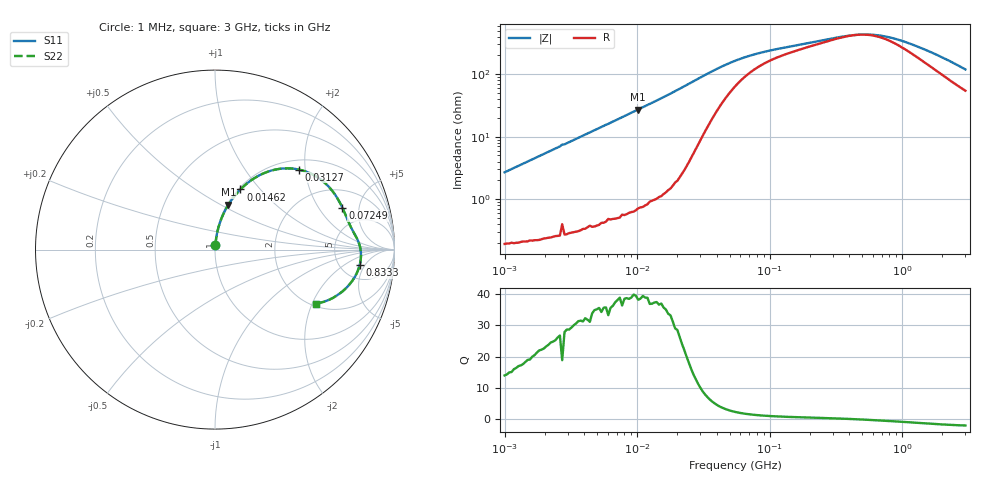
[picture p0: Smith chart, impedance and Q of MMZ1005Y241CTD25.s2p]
! S-Parameter Data Generated by TDK Corporation
! Copyright(C) 2025 TDK Corporation.
! All Rights Reserved.
! TDK P/N: MMZ1005Y241CTD25 (Chip Bead)
! Property: |Z|=240ohm at 100MHz
! Size(LxWxT): 1x0.5x0.5mm
! Model Type: s2p (Touchstone File Format Version 1.0)
! Frequency: DC=Yes Start=1MHz Stop=3000MHz 202points Log-sweep
! Model Generated on Feb. 6, 2025
! Terms and conditions regarding TDK Simulation Models:
! 1)This simulation model is being provided solely for informational
!  purposes. Please refer to the specifications of the products in
!  terms of detailed characteristics of such products.
! 2)In no event shall TDK Corporation of any of its subsidiaries be
!  liable for any loss or damage arising, directly or indirectly,
!  from any information contained in this simulation model, including,
!  but not limited to loss or damages arising from any inaccuracies,
!  omissions or errors in connection with such information.
! 3)Any and all copyrights on this simulation model are owned by
!  TDK Corporation.  Duplication or redistribution of this simulation
!  model without prior written permission from TDK Corporation
!  is prohibited.
! 4)This simulation model is subject to any modification or change
!  without any prior notice.
! 5)Neither TDK Corporation nor any of its subsidiaries shall make any
!  warranty, express or implied, including but not limited to the
!  correctness, implied warranties of merchantability and fitness for
!  a particular purpose with respect to this simulation models.
! 6)The use of this simulation model shall be deemed to have consented
!  to the terms and conditions hereof.
! Port Assignments:
!  1 ---@@@--- 2
! Applicable Conditions:
!  Temperature = 25 degC
!  DC Bias Current = 0 A
!  Small Signal Operation
# Hz S MA R 50
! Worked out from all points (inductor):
!   201 points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, 1 MHz to 3 GHz, reference 50 ohm
!   read as one part in series: L = 426 nH near 1.041 MHz
!   highest Q = 39.3 at 10.19 MHz (marker M1), where L = 425 nH
!   self-resonance near 467 MHz
!   S11 on the Smith chart (normalised r, x): 1 MHz: 1.00, +0.05; 14.62 MHz: 1.02, +0.79; 31.27 MHz: 1.21, +1.85; 72.49 MHz: 3.19, +3.37; 833.3 MHz: 7.61, -3.83; 3 GHz: 2.09, -2.12
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1000000  0.02679 84.4  0.9977 -1.5  0.9977 -1.5  0.02679 84.4
2055611  0.0547 84.4  0.9962 -3.1  0.9962 -3.1  0.0547 84.4
3900413  0.1031 82.3  0.9914 -5.9  0.9914 -5.9  0.1031 82.3
6058321  0.1575 79.2  0.9828 -9.1  0.9828 -9.1  0.1575 79.2
1.019448e7  0.2608 73.4  0.9586 -15.1  0.9586 -15.1  0.2608 73.4
1.461624e7  0.3638 67.1  0.9216 -21.3  0.9216 -21.3  0.3638 67.1
1.858443e7  0.4498 61.4  0.8788 -26.7  0.8788 -26.7  0.4498 61.4
2.362996e7  0.5453 54.1  0.8114 -33.0  0.8114 -33.0  0.5453 54.1
3.127247e7  0.6458 43.7  0.6948 -39.9  0.6948 -39.9  0.6458 43.7
4.138676e7  0.7086 33.1  0.5612 -43.6  0.5612 -43.6  0.7086 33.1
5.477226e7  0.7361 24.4  0.4488 -42.7  0.4488 -42.7  0.7361 24.4
7.248696e7  0.7472 18.2  0.3719 -38.8  0.3719 -38.8  0.7472 18.2
1.125904e8  0.759 11.9  0.3011 -31.3  0.3011 -31.3  0.759 11.9
2.136344e8  0.7824 6.4  0.239 -21.4  0.239 -21.4  0.7824 6.4
4.75755e8  0.8114 -0.2  0.1886 0.7  0.1886 0.7  0.8114 -0.2
6.049187e8  0.8141 -2.5  0.1901 10.9  0.1901 10.9  0.8141 -2.5
8.005644e8  0.8118 -5.6  0.208 22.5  0.208 22.5  0.8118 -5.6
8.332625e8  0.8107 -6.1  0.2122 24.0  0.2122 24.0  0.8107 -6.1
1.194682e9  0.7945 -10.9  0.266 34.3  0.266 34.3  0.7945 -10.9
1.645649e9  0.7643 -16.0  0.3385 38.4  0.3385 38.4  0.7643 -16.0
2.177892e9  0.7199 -21.3  0.4205 38.4  0.4205 38.4  0.7199 -21.3
3e9  0.6365 -28.3  0.5335 34.5  0.5335 34.5  0.6365 -28.3
